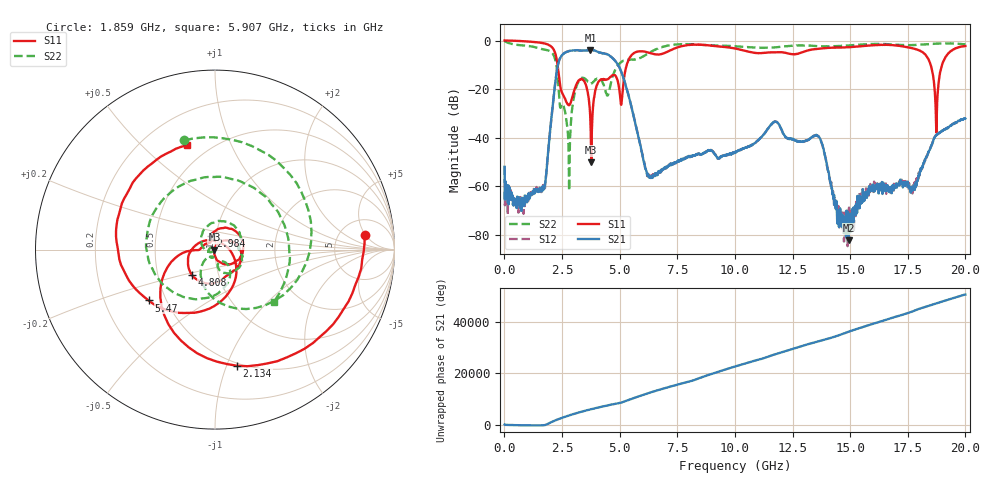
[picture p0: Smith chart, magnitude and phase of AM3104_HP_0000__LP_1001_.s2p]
!Created with skrf (http://scikit-rf.org).
# Hz S RI R 50.0
!freq ReS11 ImS11 ReS21 ImS21 ReS12 ImS12 ReS22 ImS22
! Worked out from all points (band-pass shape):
!   1601 points, 10 MHz to 20 GHz, reference 50 ohm
!   highest |S21| = -3.85 dB at 3.733 GHz (marker M1); lowest = -82.2 dB at 14.94 GHz (marker M2)
!   |S21| within 3 dB of the highest: 2.44 GHz to 4.648 GHz (2.207 GHz wide, 62.3 % of centre)
!   lowest |S11| = -50.1 dB at 3.771 GHz (marker M3), VSWR 1.01, Z = 49.7 - j0.048 ohm
!   |S11| at or under -10 dB: 2.307 GHz to 5.308 GHz (3.002 GHz wide, 78.8 % of centre); 18.49 GHz to 18.99 GHz (495 MHz wide, 2.64 % of centre)
!   |S22| runs from -61.8 to -0.2 dB; largest |S21 - S12| = 0.0054
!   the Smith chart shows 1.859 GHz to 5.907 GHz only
!   S11 on the Smith chart (normalised r, x): 1.859 GHz: 8.57, +4.80; 2.134 GHz: 0.48, -1.09; 2.984 GHz: 0.95, +0.14; 4.808 GHz: 0.75, -0.22; 5.47 GHz: 0.40, -0.29; 5.907 GHz: 0.38, +0.69
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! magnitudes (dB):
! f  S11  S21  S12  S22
! 10 MHz  0.0  -52.0  -51.8  -0.2
! 722.1 MHz  -0.2  -68.8  -65.0  -2.0
! 1.859 GHz  -1.5  -50.1  -49.8  -4.0
! 2.134 GHz  -3.6  -23.5  -23.5  -6.0
! 2.771 GHz  -26.4  -4.5  -4.4  -40.6
! 2.984 GHz  -22.0  -4.1  -4.1  -25.1
! 3.346 GHz  -15.8  -4.2  -4.2  -15.5
! 3.733 GHz  -33.5  -3.8  -3.9  -17.8
! 3.771 GHz  -50.1  -3.9  -3.9  -17.7
! 4.808 GHz  -14.4  -8.3  -8.3  -12.0
! 5.07 GHz  -26.5  -12.8  -12.8  -8.8
! 5.47 GHz  -6.6  -25.7  -25.7  -7.8
! 5.907 GHz  -4.4  -43.4  -43.4  -7.1
! 6.682 GHz  -5.8  -54.5  -54.1  -3.2
! 10.01 GHz  -3.3  -45.8  -46.2  -2.4
! 13.34 GHz  -3.7  -39.7  -39.8  -2.2
! 14.94 GHz  -2.7  -82.2  -74.3  -2.1
! 16.68 GHz  -1.8  -62.2  -61.7  -1.5
! 18.26 GHz  -5.8  -48.7  -49.0  -1.6
! 18.74 GHz  -37.9  -39.1  -38.9  -1.3
! 19.11 GHz  -7.2  -36.6  -36.6  -1.2
! 20 GHz  -2.3  -32.1  -31.9  -1.6
